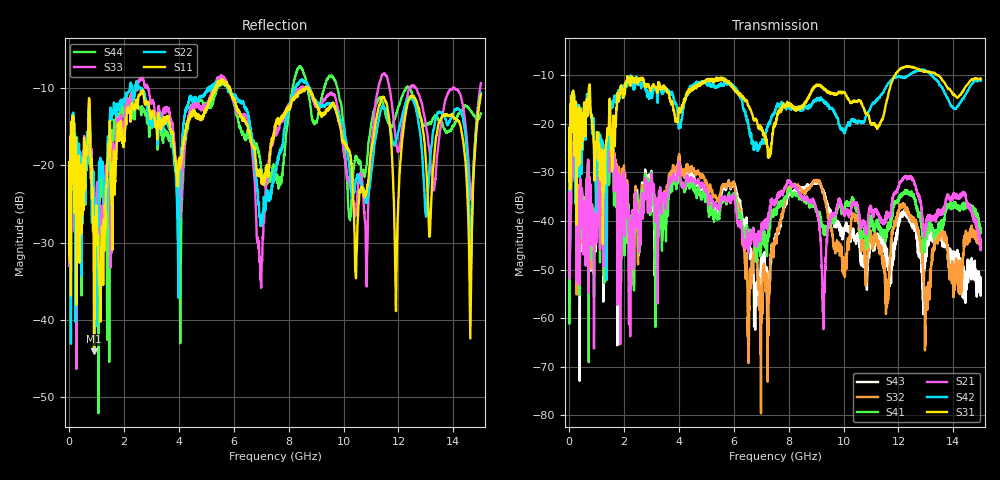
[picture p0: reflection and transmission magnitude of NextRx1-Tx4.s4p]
! FILE: N:\QM 2007\Prüfprotokolle\Highspeed\Konfektionierte Ltg\L45593-D106\D30\8216\0002\Next\NextRx1-Tx4.s4p
# MHz S DB R 50.00
! FREQ  S11  S12  S13  S14
!  S21  S22  S23  S24
!  S31  S32  S33  S34
!  S41  S42  S43  S44
!  DB  ANG  DB  ANG  DB  ANG  DB  ANG
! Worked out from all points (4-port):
!   2999 points, 10 MHz to 15 GHz, reference 50 ohm
!   strongest paths, dB at 10 MHz, 3.755 GHz, 7.505 GHz, 11.26 GHz, 15 GHz:
!     S31: -25.3, -15.3, -20.4, -20.5, -10.7
!     S42: -23.7, -13.4, -17.7, -14.9, -11.1
!     S21: -48.9, -31.7, -35.7, -38.6, -44.6
!     S41: -40.2, -33.6, -38.0, -41.7, -42.5
!     S32: -42.3, -29.6, -43.9, -44.8, -44.5
!     S43: -42.9, -31.5, -44.7, -43.5, -52.1
!   lowest |S11| = -44.1 dB at 915 MHz (marker M1), VSWR 1.01, Z = 50.6 + j0.0226 ohm
!   |S11| at or under -10 dB: start of sweep to 5.33 GHz; 5.855 GHz to 8.618 GHz (2.763 GHz wide, 38.2 % of centre); 8.711 GHz to end of sweep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
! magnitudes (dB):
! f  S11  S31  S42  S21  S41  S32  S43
! 10 MHz  -19.6  -25.3  -23.7  -48.9  -40.2  -42.3  -42.9
! 915 MHz  -44.1  -25.2  -23.5  -66.3  -55.6  -51.1  -49.5
! 5.59 GHz  -8.9  -11.0  -11.9  -35.2  -36.1  -32.8  -33.6
! 6.565 GHz  -15.6  -16.4  -20.9  -43.4  -42.6  -58.6  -44.4
! 8.17 GHz  -11.6  -16.4  -16.9  -32.7  -34.6  -32.8  -34.4
! 14.61 GHz  -41.6  -11.2  -12.2  -37.3  -37.6  -43.3  -51.5
! 15 GHz  -10.8  -10.7  -11.1  -44.6  -42.5  -44.5  -52.1
